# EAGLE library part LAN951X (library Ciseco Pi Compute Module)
LAN951X LAN9512 has two downstream USB ports LAN9514 has four downstream USB ports The same footprint is use for both but for LAN9512 (2 port) accpications the _USB1 block signals should be NC
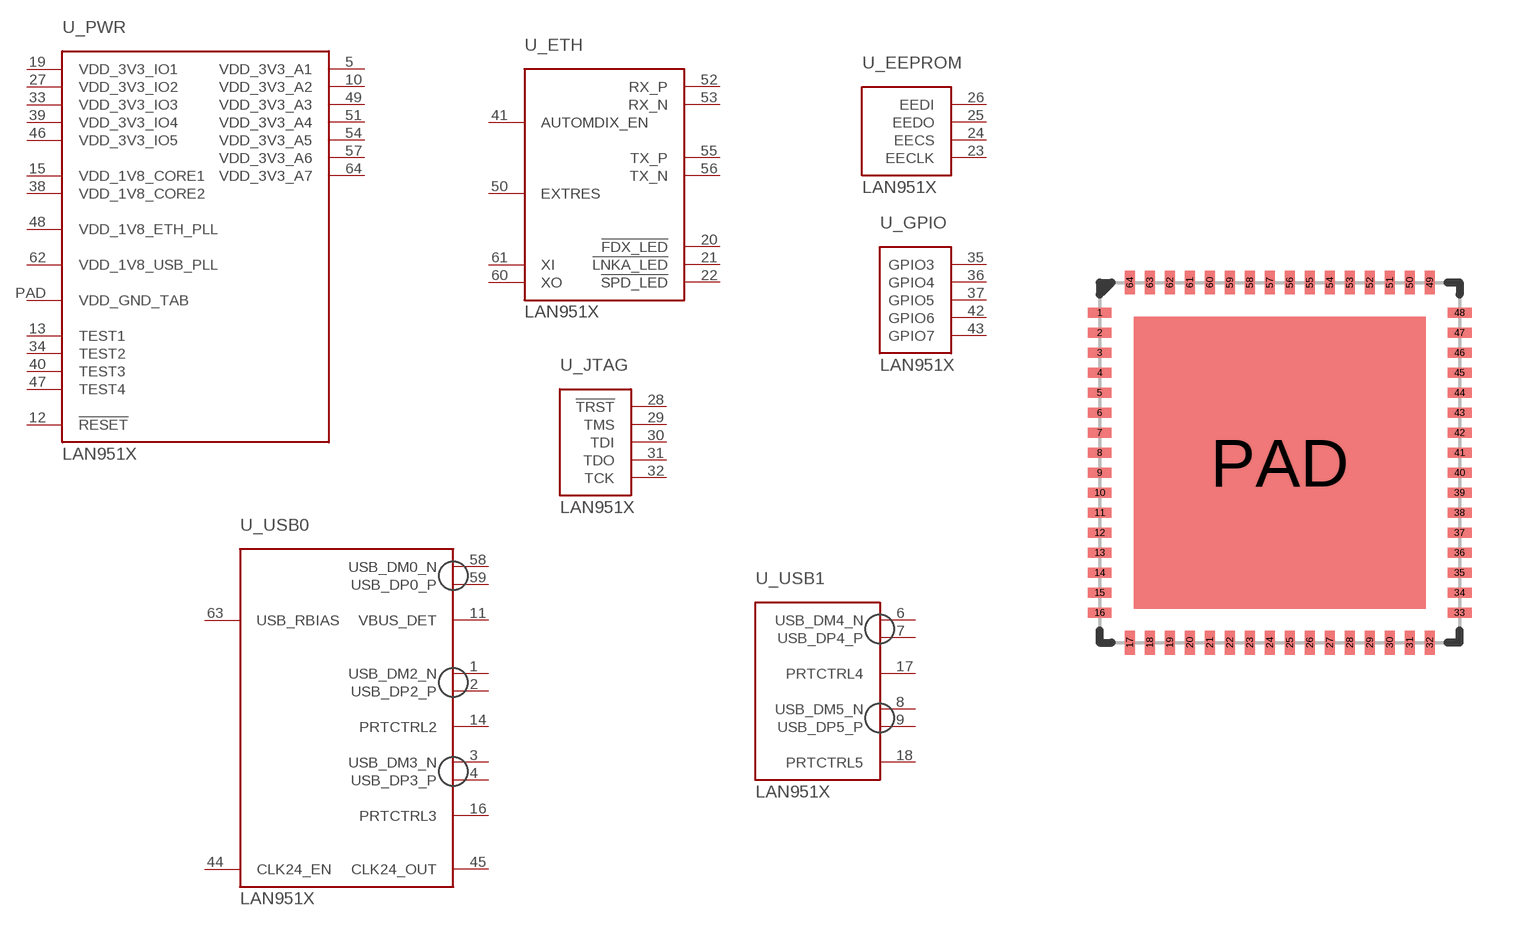
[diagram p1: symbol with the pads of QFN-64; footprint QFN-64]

Designator prefix U; gates _PWR=LAN915X_PWR _ETH=LAN915X_ETH _EEPROM=LAN915X_EEPROM _GPIO=LAN915X_GPIO _JTAG=LAN915X_JTAG _USB0=LAN915X_USB0 _USB1=LAN915X_USB1

## LAN951X  [QFN-64]
1  _USB0:USB_DM2_N
2  _USB0:USB_DP2_P
3  _USB0:USB_DM3_N
4  _USB0:USB_DP3_P
5  _PWR:VDD_3V3_A1
6  _USB1:USB_DM4_N
7  _USB1:USB_DP4_P
8  _USB1:USB_DM5_N
9  _USB1:USB_DP5_P
10  _PWR:VDD_3V3_A2
11  _USB0:VBUS_DET
12  _PWR:!RESET
13  _PWR:TEST1
14  _USB0:PRTCTRL2
15  _PWR:VDD_1V8_CORE1
16  _USB0:PRTCTRL3
17  _USB1:PRTCTRL4
18  _USB1:PRTCTRL5
19  _PWR:VDD_3V3_IO1
20  _ETH:!FDX_LED
21  _ETH:!LNKA_LED
22  _ETH:!SPD_LED
23  _EEPROM:EECLK
24  _EEPROM:EECS
25  _EEPROM:EEDO
26  _EEPROM:EEDI
27  _PWR:VDD_3V3_IO2
28  _JTAG:!TRST
29  _JTAG:TMS
30  _JTAG:TDI
31  _JTAG:TDO
32  _JTAG:TCK
33  _PWR:VDD_3V3_IO3
34  _PWR:TEST2
35  _GPIO:GPIO3
36  _GPIO:GPIO4
37  _GPIO:GPIO5
38  _PWR:VDD_1V8_CORE2
39  _PWR:VDD_3V3_IO4
40  _PWR:TEST3
41  _ETH:AUTOMDIX_EN
42  _GPIO:GPIO6
43  _GPIO:GPIO7
44  _USB0:CLK24_EN
45  _USB0:CLK24_OUT
46  _PWR:VDD_3V3_IO5
47  _PWR:TEST4
48  _PWR:VDD_1V8_ETH_PLL
49  _PWR:VDD_3V3_A3
50  _ETH:EXTRES
51  _PWR:VDD_3V3_A4
52  _ETH:RX_P
53  _ETH:RX_N
54  _PWR:VDD_3V3_A5
55  _ETH:TX_P
56  _ETH:TX_N
57  _PWR:VDD_3V3_A6
58  _USB0:USB_DM0_N
59  _USB0:USB_DP0_P
60  _ETH:XO
61  _ETH:XI
62  _PWR:VDD_1V8_USB_PLL
63  _USB0:USB_RBIAS
64  _PWR:VDD_3V3_A7
PAD  _PWR:VDD_GND_TAB

## Footprint QFN-64 (pad centres in mm)
smd 0.6 x 0.25: 1 -4.5,3.75; 2 -4.5,3.25; 3 -4.5,2.75; 4 -4.5,2.25; 5 -4.5,1.75; 6 -4.5,1.25; 7 -4.5,0.75; 8 -4.5,0.25; 9 -4.5,-0.25; 10 -4.5,-0.75; 11 -4.5,-1.25; 12 -4.5,-1.75; 13 -4.5,-2.25; 14 -4.5,-2.75; 15 -4.5,-3.25; 16 -4.5,-3.75; 33 4.5,-3.75; 34 4.5,-3.25; 35 4.5,-2.75; 36 4.5,-2.25; 37 4.5,-1.75; 38 4.5,-1.25; 39 4.5,-0.75; 40 4.5,-0.25; 41 4.5,0.25; 42 4.5,0.75; 43 4.5,1.25; 44 4.5,1.75; 45 4.5,2.25; 46 4.5,2.75; 47 4.5,3.25; 48 4.5,3.75
smd 0.25 x 0.6: 17 -3.75,-4.5; 18 -3.25,-4.5; 19 -2.75,-4.5; 20 -2.25,-4.5; 21 -1.75,-4.5; 22 -1.25,-4.5; 23 -0.75,-4.5; 24 -0.25,-4.5; 25 0.25,-4.5; 26 0.75,-4.5; 27 1.25,-4.5; 28 1.75,-4.5; 29 2.25,-4.5; 30 2.75,-4.5; 31 3.25,-4.5; 32 3.75,-4.5; 49 3.75,4.5; 50 3.25,4.5; 51 2.75,4.5; 52 2.25,4.5; 53 1.75,4.5; 54 1.25,4.5; 55 0.75,4.5; 56 0.25,4.5; 57 -0.25,4.5; 58 -0.75,4.5; 59 -1.25,4.5; 60 -1.75,4.5; 61 -2.25,4.5; 62 -2.75,4.5; 63 -3.25,4.5; 64 -3.75,4.5
smd 7.3 x 7.3: PAD 0,0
